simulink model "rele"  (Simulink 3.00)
settings: Solver=ode45  StartTime=0.0  StopTime=200  MaxStep=1  RelTol=1e-3  AbsTol=1e-3
undefined symbols (not defined in the file or in its folder): sfunyst
libraries: simulink_extras x1

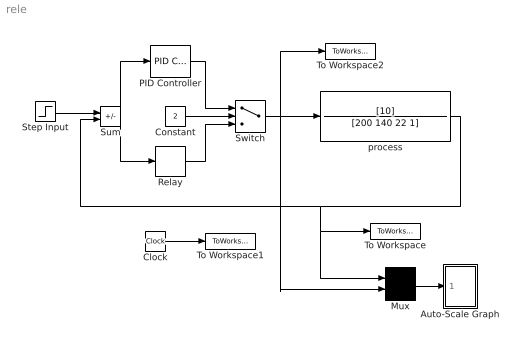
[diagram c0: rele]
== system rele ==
  Auto-Scale Graph : Subsystem  mask(Storage scope.){}
      mask help: Storage scope using MATLAB graph window. Enter plotting ranges and line type.
      mask init:
      | npts = @4; color = @5; ax = [0, @1, @2, @3]; dt=-1;
  Clock : Clock
  Constant : Constant  Value=2
  Mux : Mux  Inputs=2
  PID Controller : simulink_extras/Additional Linear/PID Controller  P=1.4  I=0.07  D=7
  Relay : Relay  OnSwitchValue=0.01  OffSwitchValue=-0.01  OnOutputValue=0.15  OffOutputValue=0.05
  Step Input : Step  Time=0  Before=0  After=1  SampleTime=1
  Sum : Sum  Inputs=+-  SaturateOnIntegerOverflow=on
  Switch : Switch  Threshold=1.5
  To Workspace : ToWorkspace  VariableName=y  SampleTime=0  SaveFormat=Matrix
  To Workspace1 : ToWorkspace  VariableName=t  SampleTime=0  SaveFormat=Matrix
  To Workspace2 : ToWorkspace  VariableName=u  SampleTime=0  SaveFormat=Matrix
  process : TransferFcn  Numerator=[10]  Denominator=[200 140 22 1]
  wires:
  Step Input/1 -> Sum/1
  process/1 -> Sum/2, To Workspace/1, Mux/1
  Clock/1 -> To Workspace1/1
  Mux/1 -> Auto-Scale Graph/1(x)
  Switch/1 -> process/1, To Workspace2/1, Mux/2
  Constant/1 -> Switch/2
  Sum/1 -> PID Controller/1, Relay/1
  PID Controller/1 -> Switch/1
  Relay/1 -> Switch/3

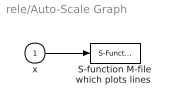
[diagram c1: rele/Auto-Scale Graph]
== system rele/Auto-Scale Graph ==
  x : Inport  Port=1  PortWidth=-1  SampleTime=-1  DataType=auto
  "S-function M-file which plots lines " : S-Function  LoadFcn=sfunyst([],[],[],'LoadBlock')  FunctionName=sfunyst  Parameters=ax, color, npts, dt  PortCounts=[]  SFunctionModules=''
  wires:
  x/1 -> "S-function M-file which plots lines "/1
